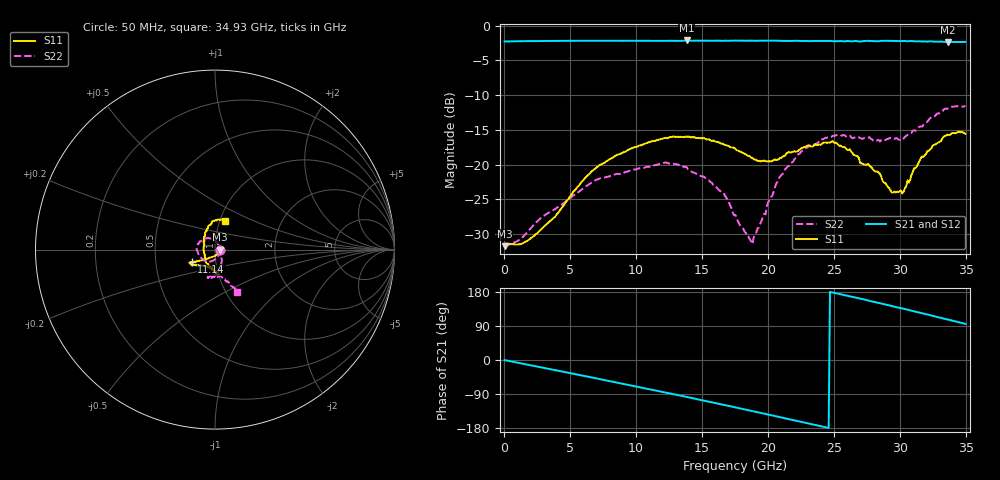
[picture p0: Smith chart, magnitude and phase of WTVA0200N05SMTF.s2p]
! 50 ohm 2-Port S-parameters measured by Modelithics Inc support@modelithics.com  Tampa, FL USA 813-866-6335 (February 2024)
! Smiths Interconnect,  2dB P/N: WTVA0200N05SMTF, Temperature: 0 C
! Board: 10 mil Rogers 4350B, Mounting Pad Dimensions: Length: 15 mils, Width: 25 mils, Gap: 40 mils.
# Hz S RI R 50
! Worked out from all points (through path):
!   352 points, 50 MHz to 34.93 GHz, reference 50 ohm
!   highest |S21| = -2.14 dB at 13.83 GHz (marker M1); lowest = -2.4 dB at 33.63 GHz (marker M2)
!   group delay of S21, straight-line fit = 21 ps
!   lowest |S11| = -31.7 dB at 50 MHz (marker M3), VSWR 1.05, Z = 52.7 - j0.0611 ohm
!   |S11| at or under -10 dB: start of sweep to end of sweep
!   |S22| runs from -31.7 to -11.6 dB; largest |S21 - S12| = 0.0052
!   S11 on the Smith chart (normalised r, x): 50 MHz: 1.05, -0.00; 11.14 GHz: 0.76, -0.11; 34.93 GHz: 1.06, +0.34
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5e7  0.0258 -0.00058  0.7689 -0.00386  0.7684 -0.00432  0.0268 -0.000461
1.195e9  0.0189 -0.0189  0.7649 -0.1075  0.7646 -0.1075  0.0214 -0.0193
2.4885e9  0.00596 -0.0313  0.74 -0.2255  0.7395 -0.2254  0.0183 -0.0342
5.8715e9  -0.0523 -0.0535  0.5911 -0.5059  0.5908 -0.5059  -0.0171 -0.0637
8.558e9  -0.0982 -0.0646  0.3939 -0.6706  0.3931 -0.6707  -0.0632 -0.0581
1.1145e10  -0.1289 -0.07  0.1593 -0.7601  0.159 -0.7599  -0.0963 -0.0159
1.1742e10  -0.1339 -0.0705  0.1022 -0.7697  0.1012 -0.7696  -0.1008 -0.00293
1.38315e10  -0.1371 -0.0803  -0.1028 -0.775  -0.1031 -0.7747  -0.084 0.0462
1.66175e10  -0.1103 -0.0861  -0.3676 -0.685  -0.3683 -0.6845  -0.0158 0.0606
1.7513e10  -0.0952 -0.088  -0.4483 -0.6385  -0.4488 -0.6379  0.00496 0.0432
1.88065e10  -0.0642 -0.0914  -0.5495 -0.5515  -0.5494 -0.5512  0.0259 0.00647
2.07965e10  -0.0124 -0.1086  -0.6745 -0.3857  -0.6746 -0.3849  0.0371 -0.0701
2.2289e10  0.0118 -0.1256  -0.7355 -0.2446  -0.7357 -0.2434  0.0226 -0.1167
2.33835e10  0.017 -0.134  -0.7634 -0.136  -0.7632 -0.1355  0.00377 -0.1365
2.4876e10  0.0175 -0.1465  -0.7712 0.0268  -0.771 0.0274  -0.0226 -0.1595
2.61695e10  0.00359 -0.1287  -0.7566 0.1617  -0.7562 0.162  -0.0402 -0.1577
2.83585e10  -0.0492 -0.0724  -0.6731 0.3775  -0.6724 0.3781  -0.0176 -0.1495
2.91545e10  -0.0574 -0.036  -0.628 0.4569  -0.627 0.4576  0.00392 -0.1544
3.01495e10  -0.0582 0.0214  -0.5574 0.5358  -0.5568 0.536  0.0276 -0.1468
3.1642e10  -0.0494 0.103  -0.4235 0.641  -0.4232 0.6408  0.0653 -0.1754
3.3632e10  0.00627 0.1632  -0.2168 0.7284  -0.2126 0.7294  0.1158 -0.2263
3.49255e10  0.056 0.1572  -0.0694 0.7602  -0.0659 0.7602  0.1222 -0.2343
